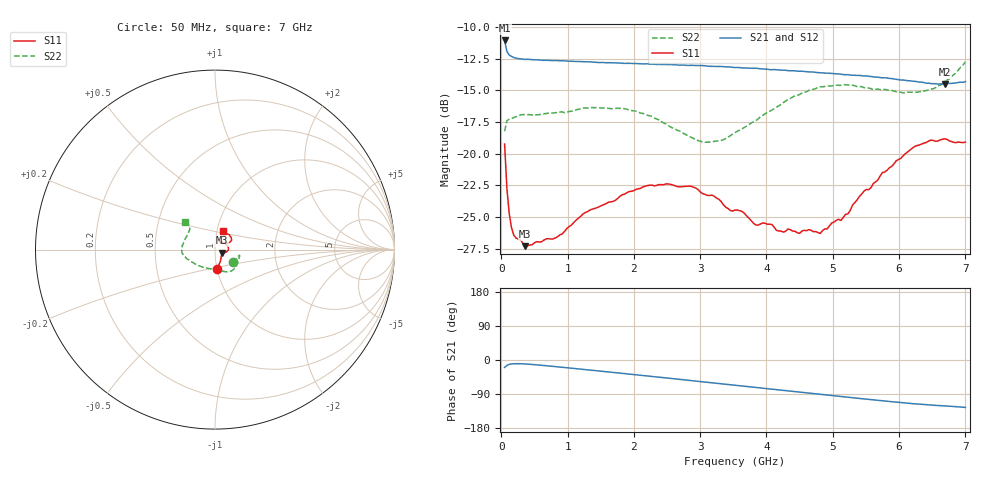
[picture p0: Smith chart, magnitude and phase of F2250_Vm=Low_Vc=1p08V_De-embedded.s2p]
! Integrated Device Technology
! Corporate Headquarters
! 6024 Silver Creek Valley Road
! San Jose, CA 95138  USA
! Phone:  1-408-284-8200
! Toll Free:  1-800-223-1366
! Webpage:  http://www.idt.com/
! Timing and RF Division
! 515 Groton Road, Suite 102
! Westford, MA 01886-6024
! Device:  F2250
! Description: Voltage Variable RF Attenuator
! Frequency:  50.0 -  6000.00 MHz
! Package:  3x3 mm Thin QFN Plastic Package: 16 pin
! Ports:  2 RF, 3 DC
!  Pin  1  = GND
!  Pin  2  = NC
!  Pin  3  = RF1  = Port 1
!  Pin  4  = NC
!  Pin  5  = GND
!  Pin  6  = GND
!  Pin  7  = GND
!  Pin  8  = GND
!  Pin  9  = NC
!  Pin 10  = RF2  = Port 2
!  Pin 11  = NC
!  Pin 12  = GND
!  Pin 13  = GND
!  Pin 14  = VCNTRL
!  Pin 15  = VDD
!  Pin 16  = VMODE
! Vcntrl:  1.080 Volts
! Vmode:  +0.000 Volts
! Vdd:  +3.30  Volts
! Current:  1.191 mA
! Data:  The device was measured on a the F2250 evaluation board which has
!  individual transmission lines to the RF pins.  Data was collected
!  using a calibrated network analyzer.  The evaluation board was
!  de-embedded using a TRL calibration technique.
!  The reference plane is the edge of the package pin.
! Misc:  SN 10
!  Action Tracker AT0258
! Date Measured:  2014-11-26
! Date:  2015-10-15  MJV
! Note:
!  Integrated Device Technology supplies this data as a sample of measured
!  data at the package pin for this product.  Your particular data for this
!  product may vary.
!  Data was taken at 25 degrees C.
!  Integrated Device Technology reserves the right to change this data at anytime.
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# GHz S dB R 50
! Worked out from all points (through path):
!   201 points, 50 MHz to 7 GHz, reference 50 ohm
!   highest |S21| = -11.07 dB at 50 MHz (marker M1); lowest = -14.5 dB at 6.687 GHz (marker M2)
!   group delay of S21, straight-line fit = 49.5 ps
!   lowest |S11| = -27.3 dB at 362.8 MHz (marker M3), VSWR 1.09, Z = 54.1 - j1.87 ohm
!   |S11| at or under -10 dB: start of sweep to end of sweep
!   |S22| runs from -19.1 to -12.8 dB; largest |S21 - S12| = 0.00059
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0.05  -19.25 -84.1  -11.07 -19.6  -11.07 -19.6  -18.24 -35.6
0.08475  -22.78 -65.7  -11.94 -14.2  -11.93 -14.1  -17.40 -19.8
0.1195  -24.73 -55.4  -12.23 -11.6  -12.21 -11.6  -17.29 -15.0
0.15425  -25.87 -47.5  -12.33 -10.4  -12.34 -10.4  -17.25 -13.6
0.189  -26.45 -40.4  -12.42 -9.9  -12.42 -9.9  -17.15 -13.2
0.36275  -27.32 -23.6  -12.57 -10.5  -12.56 -10.5  -16.93 -15.0
0.8145  -26.67 -17.1  -12.66 -17.4  -12.66 -17.4  -16.78 -28.3
1.2315  -24.78 -16.5  -12.75 -24.7  -12.75 -24.7  -16.42 -39.5
1.857  -23.21 -7.3  -12.88 -35.9  -12.87 -35.9  -16.46 -52.6
2.37825  -22.45 3.3  -12.96 -45.3  -12.95 -45.3  -17.34 -65.2
2.86475  -22.59 16.8  -13.03 -54.4  -13.03 -54.4  -18.73 -85.7
3.0385  -23.17 22.2  -13.05 -57.7  -13.06 -57.7  -19.09 -95.9
3.525  -24.47 38.6  -13.21 -66.8  -13.21 -66.8  -18.35 -126.9
3.83775  -25.64 50.5  -13.27 -72.6  -13.27 -72.6  -17.40 -142.9
4.7065  -26.17 57.0  -13.57 -88.8  -13.57 -88.8  -14.93 -171.0
4.81075  -26.31 52.5  -13.62 -90.7  -13.61 -90.7  -14.73 -172.9
5.1235  -25.28 42.5  -13.73 -96.5  -13.73 -96.5  -14.61 179.9
5.471  -22.96 31.5  -13.88 -102.6  -13.87 -102.7  -14.80 172.5
5.85325  -21.13 26.3  -14.06 -109.4  -14.06 -109.4  -15.02 162.5
6.2355  -19.43 29.9  -14.30 -115.6  -14.31 -115.7  -15.17 149.8
6.68725  -18.83 45.5  -14.52 -121.1  -14.50 -121.2  -14.33 137.4
7  -19.10 67.4  -14.32 -125.2  -14.31 -125.3  -12.76 137.3
